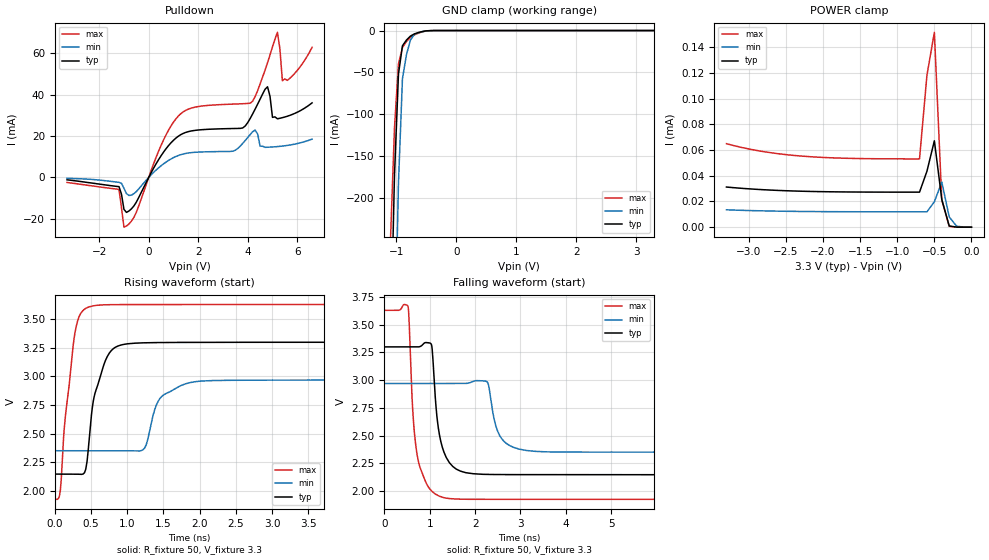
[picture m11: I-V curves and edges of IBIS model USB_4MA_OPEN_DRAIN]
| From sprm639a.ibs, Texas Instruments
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|   Model Cell USB_4MA_OPEN_DRAIN
|USB_4MA_OPEN_DRAIN
[Model]   USB_4MA_OPEN_DRAIN
Model_type   I/O_open_drain
Polarity   Inverting
Enable   Active-Low
Vinl =  0.8
Vinh =  2
Cref =  15.0000pF
Rref =  100.0000M
Vref =  0V
Vmeas =  1.65
C_comp   5.34973p   4.565931p   6.027791p
[Model Spec]
Vinl   0.8   0.8   0.8
Vinh   2   2   2
[Temperature Range]   25   155   -40
[Voltage Range]   3.3   2.97   3.63
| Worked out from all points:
|   slope of the pulldown table from 0 to 0.495 V, typ, clamps not added: 47.6 ohm
|   GND clamp passes 1 mA (typ) near -0.55 V on its own axis
|   rising waveform, R_fixture 50, V_fixture 3.3: 20-80 % time 196ps typ, 229ps min, 153ps max; typ from 2.15 V to 3.3 V
|   falling waveform, R_fixture 50, V_fixture 3.3: 20-80 % time 205ps typ, 243ps min, 183ps max; typ from 3.3 V to 2.15 V
| Nom Voltages:
|   BIASFET=3.3, VDD=1.2, VDDS=3.3, VSS=0
| Min Voltages:
|   BIASFET=2.97, VDD=1.08, VDDS=2.97, VSS=0
| Max Voltages:
|   BIASFET=3.63, VDD=1.32, VDDS=3.63, VSS=0
[POWER_clamp]
|   voltage   I(typ)   I(min)   I(max)
-3.3V     31.22uA    13.5uA     64.95uA
-2.8V     29.13uA    12.67uA    58.77uA
-2.3V     27.98uA    12.22uA    55.36uA
-1.7V     27.4uA     12.01uA    53.62uA
-700mV    27.24uA    11.95uA    53.12uA
-600mV    43.52uA    11.94uA    118.2uA
-500mV    67.21uA    19.79uA    151.6uA
-400mV    21.58uA    35.11uA    21.1uA
-300mV    927.4nA    7.959uA    611.4nA
-200mV    28.93nA    716.3nA    11.51nA
0V        696.9pA    39.48nA    568pA
[Pulldown]
|   voltage   I(typ)   I(min)   I(max)
-3.3V     -1.162mA   -442.5uA   -2.413mA
-1.2V     -4.448mA   -2.37mA    -5.833mA
-1V       -15.42mA   -5.267mA   -24.03mA
-900mV    -16.9mA    -7.758mA   -23.48mA
1.2V      19.95mA    10.62mA    29.71mA
3.4V      23.64mA    12.69mA    35.45mA
4.1V      28.51mA    20.74mA    35.87mA
4.8V      43.85mA    14.6mA     55.43mA
5V        29.04mA    14.73mA    63.13mA
5.2V      28.35mA    14.92mA    70.15mA
5.4V      28.9mA     15.16mA    46.73mA
6.6V      36.05mA    18.53mA    62.9mA
[GND_clamp]
|   voltage   I(typ)   I(min)   I(max)
-3.3V     -16.36A    -15.08A    -17.18A
-1.1V     -382.1mA   -717.8mA   -250.1mA
-1.033V   -173.3mA   -402.2mA   -116.4mA
-966.7mV  -52.02mA   -182.1mA   -39.81mA
-900mV    -18.21mA   -57.43mA   -20.34mA
-833.3mV  -11.36mA   -28.88mA   -13.17mA
-766.7mV  -6.618mA   -11.27mA   -8.134mA
-700mV    -3.983mA   -4.59mA    -5.247mA
-500mV    -328.3uA   -481.4uA   -374.5uA
-366.7mV  -15.94uA   -50.74uA   -14.83uA
3.3V      696.9pA    15.85uA    426.1pA
[Ramp]
| variable   typ   min   max
dV/dt_f 0.71606892/0.20269188n 0.38743512/0.24185261n  1.0546967/0.18146274n
dV/dt_r 0.91898113/0.19572134n 0.57962754/0.28813413n  1.2382929/0.16793875n
R_load = 50
[Rising Waveform]
R_fixture = 50
V_fixture = 3.3
V_fixture_min = 2.97
V_fixture_max = 3.63
|   time   V(typ)   V(min)   V(max)
0s        2.146V     2.35V      1.925V
76.7ps    2.146V     2.35V      2.003V
138ps     2.146V     2.35V      2.597V
294.6ps   2.145V     2.35V      3.436V
427.5ps   2.188V     2.35V      3.596V
566.9ps   2.877V     2.35V      3.622V
864.2ps   3.265V     2.35V      3.629V
1.497ns   3.297V     2.836V     3.63V
2.101ns   3.299V     2.963V     3.63V
20.04ns   3.3V       2.97V      3.63V
[Falling Waveform]
R_fixture = 50
V_fixture = 3.3
V_fixture_min = 2.97
V_fixture_max = 3.63
|   time   V(typ)   V(min)   V(max)
0s        3.3V       2.97V      3.63V
518.5ps   3.3V       2.97V      3.665V
694.4ps   3.3V       2.97V      2.396V
1.031ns   3.325V     2.97V      2.004V
1.17ns    2.625V     2.97V      1.961V
1.326ns   2.337V     2.97V      1.938V
2.257ns   2.15V      2.986V     1.925V
2.586ns   2.148V     2.471V     1.925V
3.326ns   2.147V     2.358V     1.925V
20.04ns   2.146V     2.35V      1.925V
